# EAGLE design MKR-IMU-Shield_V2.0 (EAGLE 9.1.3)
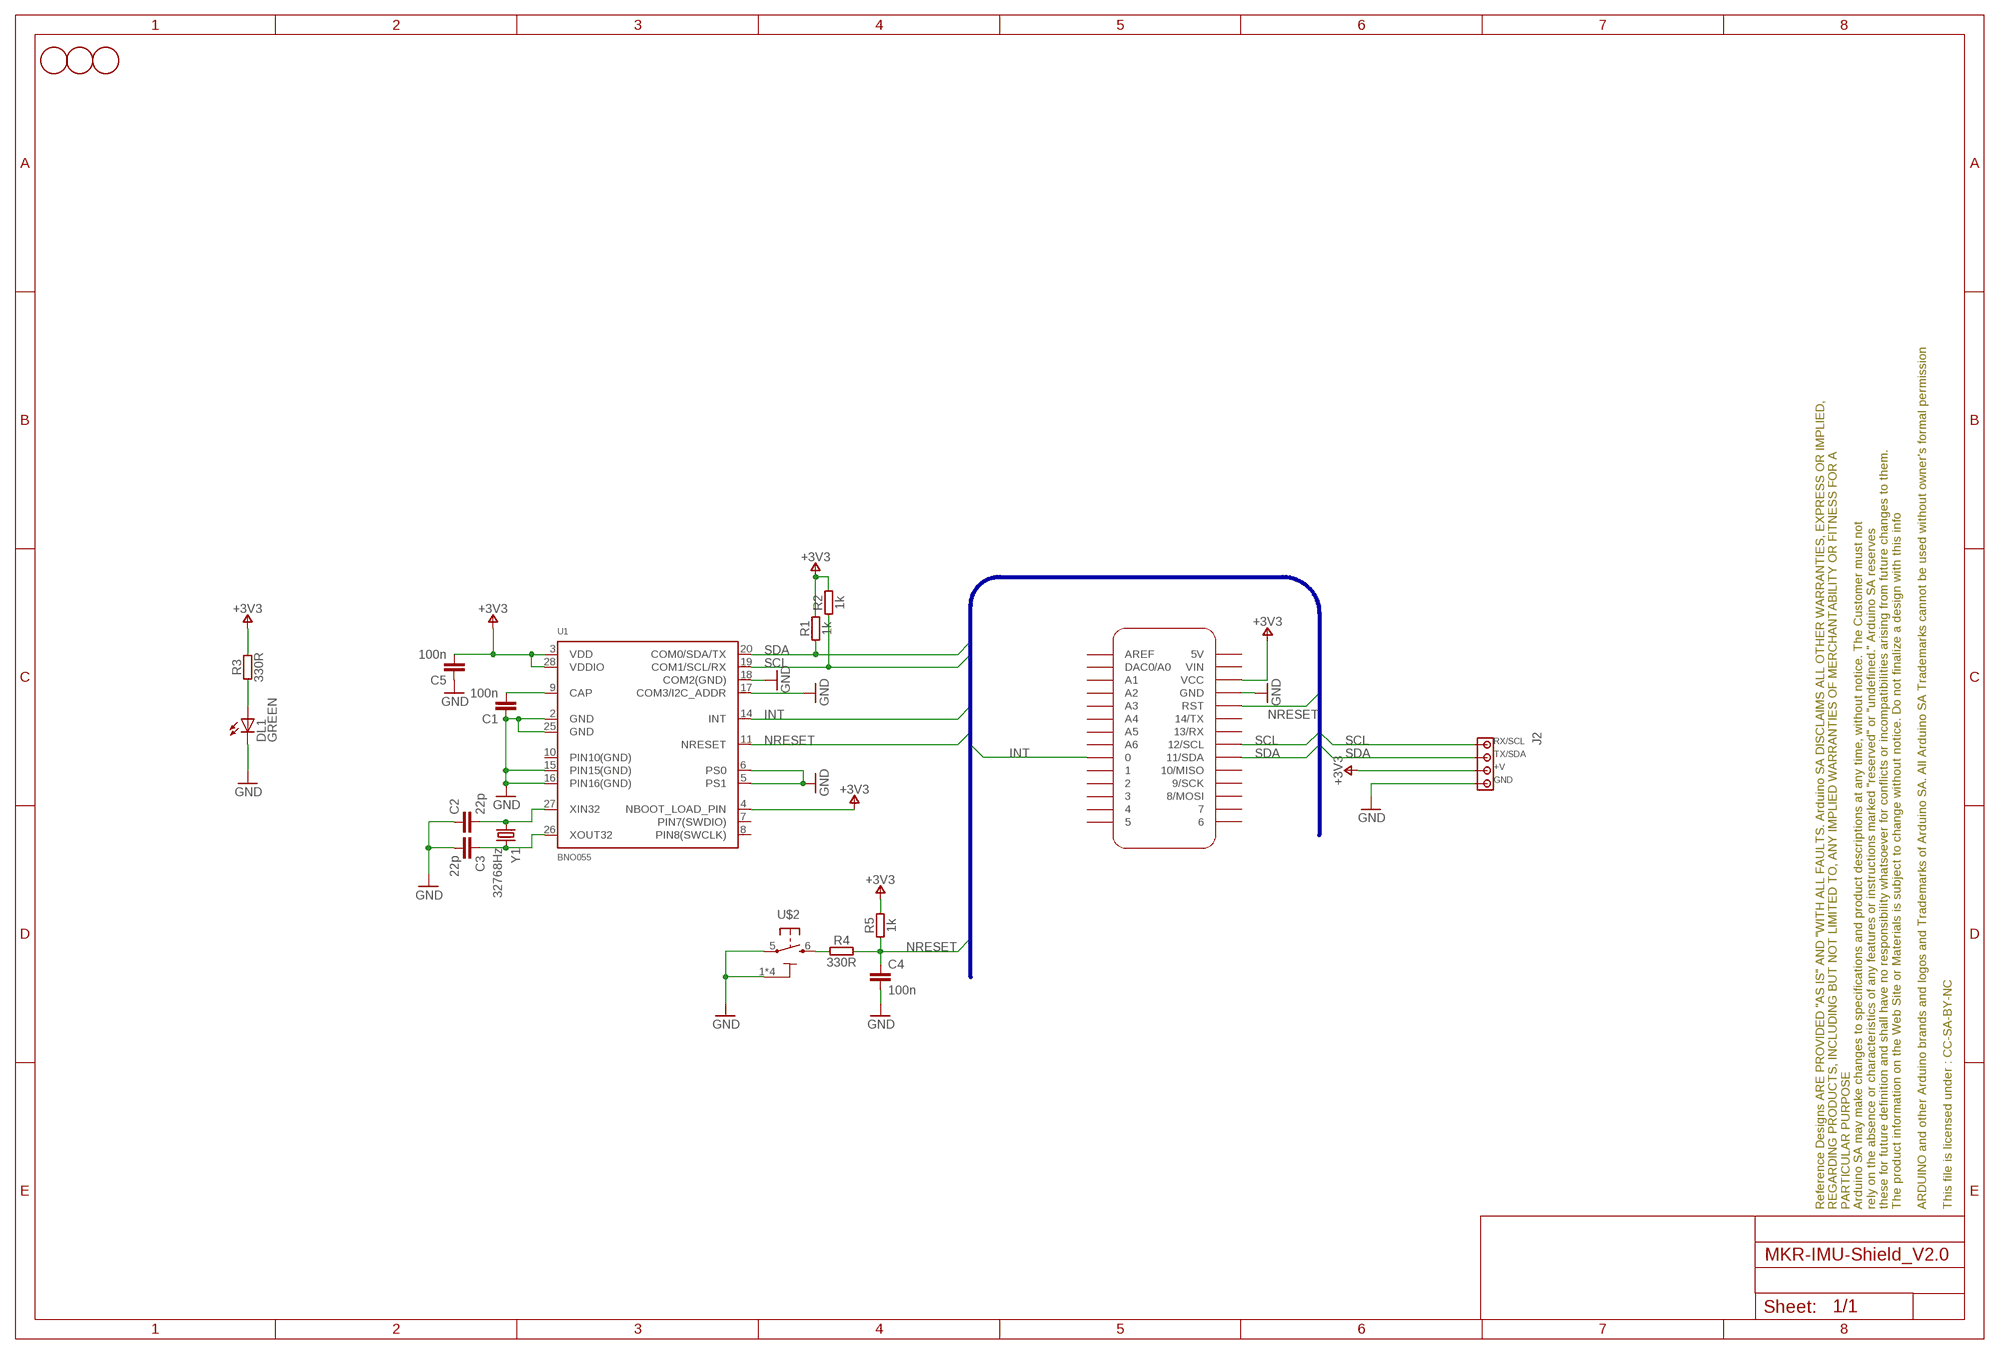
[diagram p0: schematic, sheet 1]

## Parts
C1  100n  C-100NF-0402  [0402-1005X55N]
C2  22p  C-22PF-0402  [0402-1005X55N]
C3  22p  C-22PF-0402  [0402-1005X55N]
C4  100n  C-100NF-0402  [0402-1005X55N]
C5  100n  C-100NF-0402  [0402-1005X55N]
DL1  GREEN  LED-GREEN-0603  [LEDC1608X80N-AK]
FD1  DNP  FIDUCIAL-1.5MM  [FD-1-1.5]
FD2  DNP  FIDUCIAL-1.5MM  [FD-1-1.5]
FD3  DNP  FIDUCIAL-1.5MM  [FD-1-1.5]
FRAME1  DNP  A3-FRAME-STANDARD  [FRAME]
J2  MODULINO-4RA  [MODULINO-4-RA]
MKR1  DNP  MKRBOARDOUTLINE  [MKRBOARD]
R1  1k  R-1K-0402  [0402-1005X55N]
R2  1k  R-1K-0402  [0402-1005X55N]
R3  330R  R-330R-0402  [0402-1005X55N]
R4  330R  R-330R-0402  [0402-1005X55N]
R5  1k  R-1K-0402  [0402-1005X55N]
U1  BNO055  [BNO055]
U$2  PTS820  TACTILE1PTS820-NH  [C&K_PTS820_NO_HOLES]
Y1  32768Hz  32.768KHZ  [ABS07]

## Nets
+3V3: C5.2 J2.P$3 MKR1.VCC R1.2 R2.2 R3.2 R5.2 U1.3(VDD) U1.4(NBOOT_LOAD_PIN) U1.28(VDDIO)
GND: C1.1 C2.1 C3.2 C4.2 C5.1 DL1.C J2.P$4 MKR1.GND U1.2(GND) U1.5(PS1) U1.6(PS0) U1.15(PIN15(GND)) U1.16(PIN16(GND)) U1.17(COM3/I2C_ADDR) U1.18(COM2(GND)) U1.25(GND) U$2.1 U$2.2 U$2.3 U$2.4 U$2.5
INT: MKR1.0 U1.14(INT)
N$1: DL1.A R3.1
N$2: R4.1 U$2.6
N$3: C1.2 U1.9(CAP)
N$5: C2.2 U1.27(XIN32) Y1.1
N$6: C3.1 U1.26(XOUT32) Y1.2
NRESET: C4.1 MKR1.RST R4.2 R5.1 U1.11(NRESET)
SCL: J2.P$1 MKR1.12(12/SCL) R2.1 U1.19(COM1/SCL/RX)
SDA: J2.P$2 MKR1.11(11/SDA) R1.1 U1.20(COM0/SDA/TX)
Unconnected: MKR1.1 MKR1.2 MKR1.3 MKR1.4 MKR1.5 MKR1.5V MKR1.6 MKR1.7 MKR1.8(8/MOSI) MKR1.9(9/SCK) MKR1.10(10/MISO) MKR1.13(13/RX) MKR1.14(14/TX) MKR1.A0(DAC0/A0) MKR1.A1 MKR1.A2 MKR1.A3 MKR1.A4 MKR1.A5 MKR1.A6 MKR1.AREF MKR1.VIN U1.7(PIN7(SWDIO)) U1.8(PIN8(SWCLK)) U1.10(PIN10(GND))

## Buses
SDA,SCL,NBOOT,INT,NRESET

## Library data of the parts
C1 C4 C5 = Arduino-rcl:C: SMD Capacitor; DATASHEET: http://www.tdk.com/pdf/TDKMLCCCapRange.pdf; DISTRIBUTOR-LINK: http://www.digikey.com/product-detail/en/tdk-corporation/C1005X5R1H104K050BB/445-5942-1-ND/2443982; DISTRIBUTOR-PN: 445-5942-1-ND; MANUFACTURER: TDK; MANUFACTURER-PN: C1005X5R1H104K050BB
C2 C3 = Arduino-rcl:C: SMD Capacitor; DATASHEET: http://search.murata.co.jp/Ceramy/image/img/A01X/partnumbering_e_01.pdf; DISTRIBUTOR-LINK: https://www.digikey.se/products/en?keywords=490-8589-1-ND; DISTRIBUTOR-PN: 490-8589-1-ND; MANUFACTURER: Murata; MANUFACTURER-PN: GRM1555C1H220FA01D
DL1 = Arduino-diodes:LED: LED; DATASHEET: http://media.digikey.com/pdf/Data%20Sheets/Avago%20PDFs/HSMz-Czzz.pdf; DISTRIBUTOR-LINK: http://www.digikey.com/product-detail/en/broadcom-limited/HSMG-C190/516-1425-1-ND/637749; DISTRIBUTOR-PN: 516-1425-1-ND; MANUFACTURER: Avago; MANUFACTURER-PN: HSMG-C190
FD1-FD3 = Arduino-utility:FIDUCIAL: Fiducial mount; CODE-ARDUINO: DNP; DATASHEET: DNP; DISTRIBUTOR-LINK: DNP; DISTRIBUTOR-PN: DNP; MANUFACTURER: DNP; MANUFACTURER-PN: DNP
FRAME1 = Arduino-utility:A3-FRAME: Schematic frame; CODE-ARDUINO: DNP; DATASHEET: DNP; DISTRIBUTOR-LINK: DNP; DISTRIBUTOR-PN: DNP; MANUFACTURER: DNP; MANUFACTURER-PN: DNP
J2 = Arduino-connectors:MODULINO-4: Modulino 4 connector
MKR1 = Arduino-utility:MKRBOARD: MKR board footprint; DATASHEET: DNP; DISTRIBUTOR-LINK: DNP; DISTRIBUTOR-PN: DNP; MANUFACTURER: DNP; MANUFACTURER-PN: DNP
R1 R2 R5 = Arduino-rcl:R: SMD Resistor; DATASHEET: www.yageo.com.tw/exep/pages/download/literatures/PYu-R_INT-thick_7.pdf; DISTRIBUTOR-LINK: http://www.digikey.com/product-detail/en/yageo/RC0402FR-071KL/311-1.00KLRCT-ND/729460; DISTRIBUTOR-PN: 311-1.00KLRCT-ND; MANUFACTURER: Yageo; MANUFACTURER-PN: RC0402FR-071KL
R3 R4 = Arduino-rcl:R: SMD Resistor; DATASHEET: www.yageo.com.tw/exep/pages/download/literatures/PYu-R_INT-thick_7.pdf; DISTRIBUTOR-LINK: http://www.digikey.com/product-detail/en/yageo/RC0402FR-07330RL/311-330LRCT-ND/729541; DISTRIBUTOR-PN: 311-330LRCT-ND; MANUFACTURER: Yageo; MANUFACTURER-PN: RC0402FR-07330RL
U1 = Arduino-Sensors:BNO055: BNO055 - Motion Co-Processor; CODE-BCE: -; CODE-TK2: -; DATASHEET: https://ae-bst.resource.bosch.com/media/_tech/media/datasheets/BST_BNO055_DS000_14.pdf; DISTRIBIUTOR-PN: 828-1058-1-ND; DISTRIBUTOR-LINK: http://www.digikey.it/product-detail/it/bosch-sensortec/BNO055/828-1058-1-ND/6136309; MANUFACTURER: Bosch Sensortec; MANUFACTURER-PN: BNO055
U$2 = Arduino-pushbuttons:TACTILE1: Tactile Switch SPST-NO Top Actuated Surface Mount; DATASHEET: http://www.ckswitches.com/media/1474/pts820.pdf; DISTRIBUTOR-LINK: https://www.digikey.com/product-detail/en/c-k/PTS820-J15M-SMTR-LFS/CKN10506CT-ND/4176681; DISTRIBUTOR-PN: PTS820 J25K SMTR LFS-ND; MANUFACTURER: C&K; MANUFACTURER-PN: PTS820 J25K SMTR LFS
Y1 = Arduino-crystals:32.768KHZ: LF crystal; CODE-BCE: -; CODE-TK2: -; DATASHEET: http://www.abracon.com/Resonators/ABS07.pdf; DISTRIBUTOR-LINK: http://www.digikey.com/product-detail/en/abracon-llc/ABS07-32.768KHZ-T/535-9542-1-ND/1237009; DISTRIBUTOR-PN: 535-9542-1-ND; MANUFACTURER: Abracon LLC; MANUFACTURER-PN: ABS07-32.768KHZ-T

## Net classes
0 default: width 0.25 mm, drill 0.25 mm

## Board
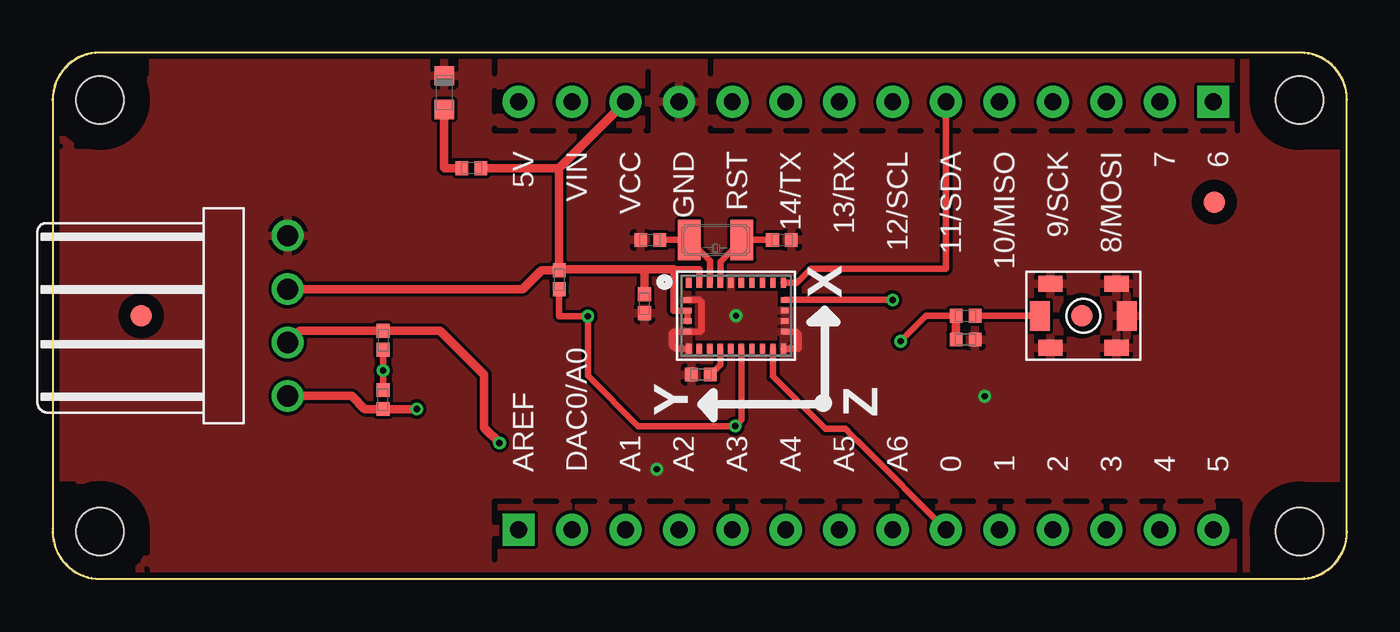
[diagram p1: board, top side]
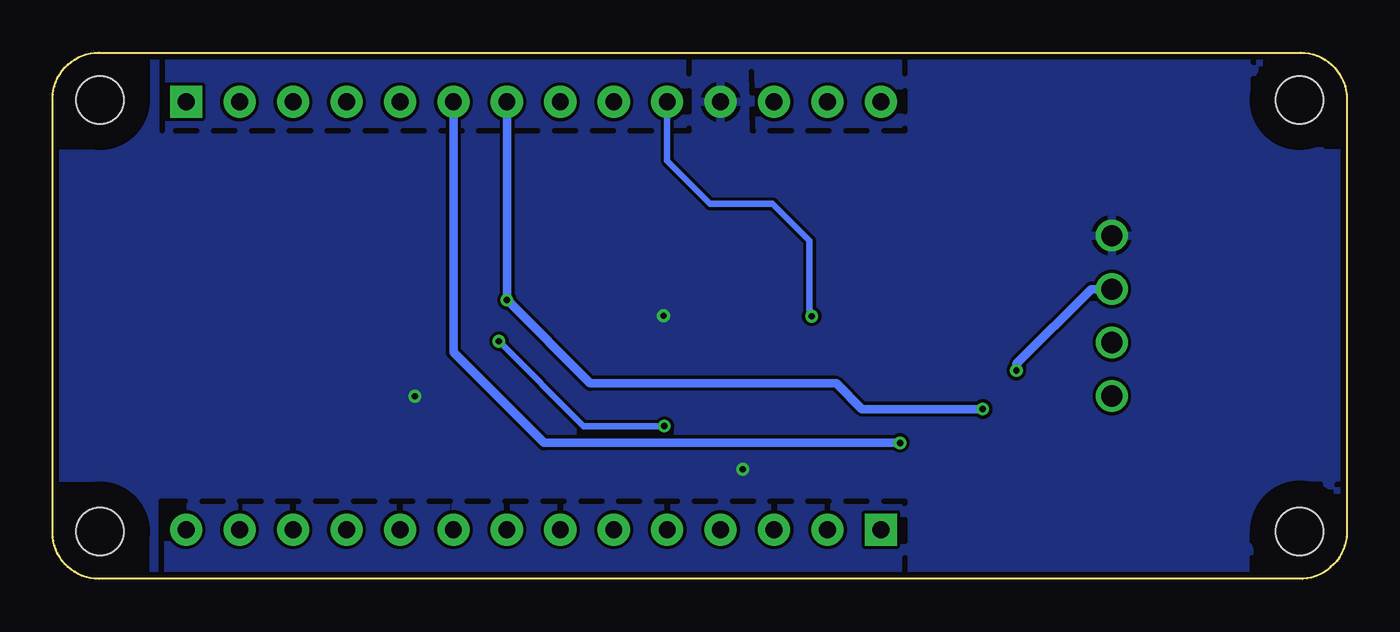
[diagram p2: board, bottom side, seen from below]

Size 61.5 x 25 mm. Coordinates in mm from the lower left corner, seen from the top.
Outline: 0,22.8 0,2.4 arc90 2.1,0 59.3,0 arc90 61.5,2.2 61.5,22.8 arc90 59.3,25 2.2,25 arc90 0,22.8
Copper layers (1*16): Top 0.035mm / dielectric 1.5mm / Bottom 0.035mm
Design rules "SeeedStudio_2layers *": minimum track width 6mil, minimum drill 0.29971875mm, track to track 6mil, track to pad 6mil, pad to pad 6mil, via to via 6mil, smd to smd 0mil, copper to edge 10mil, drill to drill 10mil, minimum pad ring 10mil, minimum via ring 6mil, stop-mask expansion 2mil, vias tented up to drill 100mil, thermal gap 8mil
tRestrict: area 0,20.5 to 4.5,25; area 57,20.5 to 61.5,25; area 57,0 to 61.5,4.5; area 0,0 to 4.5,4.5; 110 lines
bRestrict: area 0,20.5 to 4.5,25; area 57,0 to 61.5,4.5; area 57,20.5 to 61.5,25; area 0,0.1 to 4.5,4.5; 113 lines

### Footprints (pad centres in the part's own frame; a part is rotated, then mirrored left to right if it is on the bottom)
0402-1005X55N = smd 0.62 x 0.62: 1 -0.45,0; 2 0.45,0
LEDC1608X80N-AK = smd 0.9 x 0.95: A 0.8,0; C -0.8,0
FD-1-1.5 = smd 1.016 x 1.016: P$1 0,0
MODULINO-4-RA = drill 1: P$1 -3.81,-1.27; P$2 -1.27,-1.27; P$3 1.27,-1.27; P$4 3.81,-1.27
MKRBOARD = drill 0.8 pad 1.524: 0 42.455,2.34; 1 44.995,2.34; 2 47.535,2.34; 3 50.075,2.34; 4 52.615,2.34; 5 55.155,2.34; 5V 22.135,22.66; 7 52.615,22.66; 8 50.075,22.66; 9 47.535,22.66; 10 44.995,22.66; 11 42.455,22.66; 12 39.915,22.66; 13 37.375,22.66; 14 34.835,22.66; A0 24.675,2.34; A1 27.215,2.34; A2 29.755,2.34; A3 32.295,2.34; A4 34.835,2.34; A5 37.375,2.34; A6 39.915,2.34; GND 29.755,22.66; RST 32.295,22.66; VCC 27.215,22.66; VIN 24.675,22.66 | drill 0.8 pad 1.524 square: 6 55.155,22.66; AREF 22.135,2.34 | hole 2.25: 59.25,2.25; 59.25,22.75; 2.25,2.25; 2.25,22.75
BNO055 = smd 0.25 x 0.475: 1 -2.25,1.562; 6 -2.25,-1.562; 7 -1.75,-1.562; 8 -1.25,-1.562; 9 -0.75,-1.562; 10 -0.25,-1.562; 11 0.25,-1.562; 12 0.75,-1.562; 13 1.25,-1.562; 14 1.75,-1.562; 15 2.25,-1.562; 20 2.25,1.562; 21 1.75,1.562; 22 1.25,1.562; 23 0.75,1.562; 24 0.25,1.562; 25 -0.25,1.562; 26 -0.75,1.562; 27 -1.25,1.562; 28 -1.75,1.562 | smd 0.375 x 0.25: 2 -2.312,0.75; 3 -2.312,0.25; 4 -2.312,-0.25; 5 -2.312,-0.75; 16 2.312,-0.75; 17 2.312,-0.25; 18 2.312,0.25; 19 2.312,0.75
C&K_PTS820_NO_HOLES = smd 1.15 x 0.75: 1 -1.575,1.525; 2 -1.575,-1.525; 3 1.575,1.525; 4 1.575,-1.525 | smd 0.95 x 1.4: 5 -2.075,0; 6 2.075,0
ABS07 = smd 1.1 x 1.9: 1 -1.25,0; 2 1.25,0

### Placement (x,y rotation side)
C1  30.8,9.71 0 top
C2  28.39,16.1 0 top
C3  34.65,16.1 0 top
C4  43.38,11.37 0 top
C5  28.12,13.07 90 top
DL1  18.61,23.1 270 top
FD1  4.2,12.5 0 top
FD2  55.2,17.9 0 top
FD3  48.9,12.5 0 top
FRAME1  not placed on the board
J2  9.9,12.5 90 top
MKR1  0,0 0 top
R1  15.71,11.34 270 top
R2  15.7,8.52 90 top
R3  19.9,19.51 0 top
R4  43.38,12.5 180 top
R5  24.07,14.21 90 top
U1  32.48,12.5 0 top
U$2  48.98,12.5 180 top
Y1  31.5,16.1 0 top

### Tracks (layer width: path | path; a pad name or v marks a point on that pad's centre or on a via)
+3V3  (via drill 0.3)
  Top 0.305: R1.2 v15.7,9.9 R2.2 | U1.4 U1.3 29.5,12.75 29.5,14.7 30.73,14.7 U1.28 | R3.2
  Top 0.406: MKR1.VCC 24.07,19.52 | 24.07,19.52 R3.2 | C5.2 28.12,14.7 | 24.07,19.52 R5.2 | 29.5,14.7 28.12,14.7 | 28.12,14.7 24.07,14.7 R5.2 | R5.2 23.22,14.66 22.32,13.76 22.31,13.77 J2.P$3
  Bottom 0.406: v15.7,9.9 15.7,10.21 12.14,13.77 J2.P$3
GND  (via drill 0.3)
  Top 0.305: U1.16 35.34,11.75 35.45,11.64 35.45,10.96 35.43,10.94 U1.15 | U1.2 30.74,13.25 30.82,13.17 30.82,11.78 30.79,11.75 U1.5 29.5,11.75 29.44,11.69 29.44,11.11 29.62,10.94 U1.6
  other vias: 32.47,12.5 28.7,5.21 44.29,8.68
  pour Top: 0.18,24.98 61.35,25.05 61.4,0.12 0.05,0.1
  pour Bottom: 0.18,24.9 0,0.05 61.4,0.12 61.4,25.07 0.23,25
INT
  Top 0.305: MKR1.0 38.38,6.42 37.99,6.81 37.67,7.13 36.72,7.13 34.23,9.62 U1.14
N$1
  Top 0.305: 18.63,19.51 18.61,19.53
  Top 0.406: DL1.A 18.61,19.53 | R3.1 18.63,19.51
N$2
  Top 0.305: U$2.6 R4.1
N$3
  Top 0.305: U1.9 31.73,10.19 C1.2
N$5
  Top 0.305: C2.2 Y1.1 31.23,15.12 U1.27
N$6
  Top 0.305: C3.1 Y1.2 31.73,15.07 U1.26
NRESET  (via drill 0.3)
  Top 0.305: R5.1 24.07,12.48 v25.43,12.48 25.43,9.64 27.81,7.26 v32.43,7.26 32.73,7.55 U1.11 | R4.2 41.5,12.5 v40.29,11.29
  Top 0.406: C4.1 R4.2
  Bottom 0.305: MKR1.RST 32.3,19.86 30.25,17.82 27.29,17.82 25.53,16.06 25.53,12.58 v25.43,12.48 | v40.29,11.29 36.26,7.26 v32.43,7.26
SCL  (via drill 0.3)
  Top 0.305: U1.19 v39.91,13.25
  Top 0.406: v17.3,8.07 R2.1 14.83,8.07 14.21,8.69 J2.P$1
  Bottom 0.305: v39.92,13.25 v39.91,13.25
  Bottom 0.406: MKR1.12 v39.92,13.25 | v17.3,8.07 23.04,8.07 24.26,9.29 35.95,9.29 v39.91,13.25
SDA  (via drill 0.3)
  Top 0.305: U1.20 35.37,14.06 36.03,14.73 42.46,14.73 MKR1.11 | R1.1
  Top 0.406: v21.23,6.46 20.5,7.19 20.5,9.7 18.42,11.79 R1.1 12,11.79 11.76,11.79 11.73,11.79 J2.P$2
  Bottom 0.305: MKR1.11
  Bottom 0.406: v21.23,6.46 38.15,6.46 42.46,10.77 MKR1.11

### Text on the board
tPlace: X | Y | Z

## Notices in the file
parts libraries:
Arduino-utility: This file is licensed under : CC-SA-BY-NC
Arduino-Sensors: Copyright (c) 2016-2017 Arduino LLC. All right reserved.
